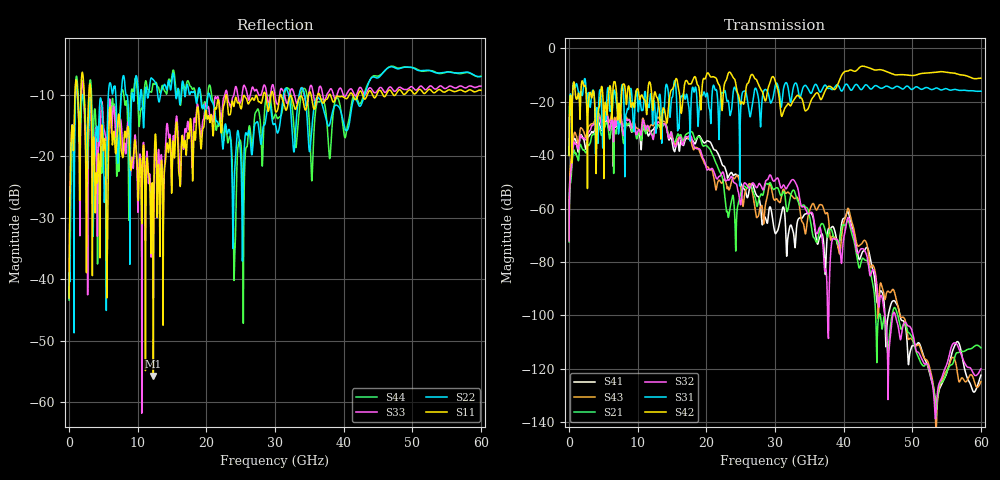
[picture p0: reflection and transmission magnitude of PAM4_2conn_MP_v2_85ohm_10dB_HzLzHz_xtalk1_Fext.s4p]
! Info: Touchstone file created by Circ.  Input file=FAB50GbE_2conn_Midplane_Examax_Topo2_v2_85ohm_10dB_HzLzHz.circ
# Hz S RI R 50
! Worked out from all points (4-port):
!   6000 points, 10 MHz to 60 GHz, reference 50 ohm
!   strongest paths, dB at 10 MHz, 15.01 GHz, 30.01 GHz, 45.01 GHz, 60 GHz:
!     S42: -40.1, -15.4, -12.0, -8.0, -11.2
!     S31: -39.8, -18.3, -14.3, -14.3, -16.0
!     S32: -72.1, -32.8, -49.4, -94.2, -120.0
!     S21: -72.5, -32.0, -52.5, -102.7, -112.1
!     S43: -71.2, -33.3, -56.7, -99.2, -124.7
!     S41: -67.6, -34.8, -69.1, -94.7, -122.4
!   lowest |S11| = -55.7 dB at 12.28 GHz (marker M1), VSWR 1.00, Z = 50 + j0.163 ohm
!   |S11| at or under -10 dB: 3.186 GHz to 22.88 GHz (19.69 GHz wide, 151 % of centre); 22.91 GHz to 28.29 GHz (5.382 GHz wide, 21 % of centre); 30.86 GHz to 34.89 GHz (4.029 GHz wide, 12.3 % of centre)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
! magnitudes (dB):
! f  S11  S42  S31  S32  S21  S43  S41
! 10 MHz  -43.0  -40.1  -39.8  -72.1  -72.5  -71.2  -67.6
! 1.11 GHz  -7.9  -19.1  -13.2  -36.2  -40.1  -33.1  -36.1
! 12.28 GHz  -55.7  -20.5  -22.1  -34.0  -33.0  -28.9  -30.4
! 24.12 GHz  -11.2  -11.5  -14.5  -50.3  -62.0  -48.8  -47.2
! 32.75 GHz  -11.7  -19.3  -14.0  -49.3  -53.1  -56.1  -70.1
! 37.44 GHz  -10.8  -15.3  -14.0  -83.1  -69.0  -61.9  -78.8
! 60 GHz  -9.3  -11.2  -16.0  -120.0  -112.1  -124.7  -122.4
